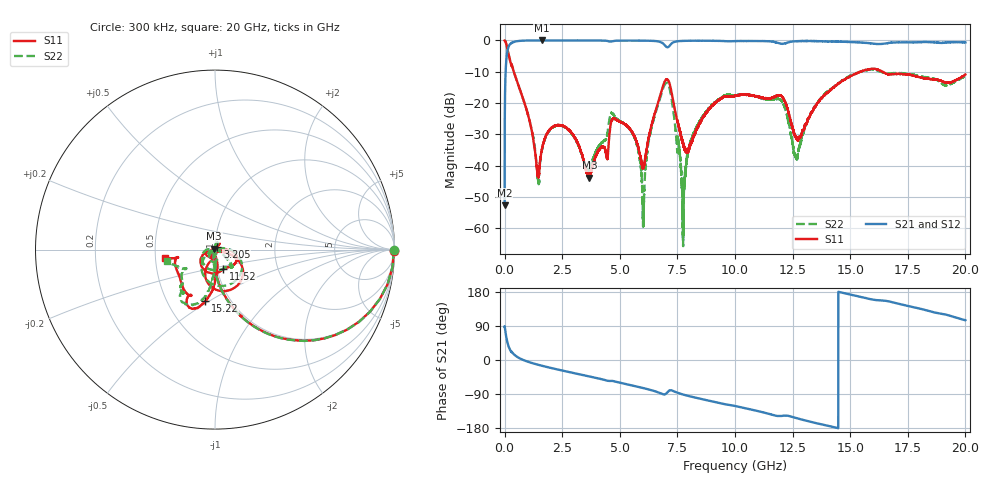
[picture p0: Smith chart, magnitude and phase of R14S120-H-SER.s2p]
!{R14S120}
!Johanson Technology Inc.
!www.johansontechnology.com
!Test Board Conditions:
!Substrate Type  RO4350B
!Substrate Thickness  20 mil
!Substrate Dk  3.66
!TL Type: GCPW
!TL Trace Width  36 mil
!TL Gap  12 mil
!Electrode orientation  Horizontal
!DUT TOPOLOGY	SERIES
!Mounting Pad LxW  26x36 mil
! Created Wed Nov 25 17:33:21 2020
! 2 Port Network Data from SP1.SP block
! freq  magS11  angS11  magS21  angS21  magS12  angS12  magS22  angS22
# khz S ma R 50
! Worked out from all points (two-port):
!   20001 points, 300 kHz to 20 GHz, reference 50 ohm
!   highest |S21| = 0.00 dB at 1.611 GHz (marker M1); lowest = -52.6 dB at 300 kHz (marker M2)
!   |S21| within 3 dB of the highest: 133.4 MHz to end of sweep
!   lowest |S11| = -43.9 dB at 3.683 GHz (marker M3), VSWR 1.01, Z = 49.6 + j0.485 ohm
!   |S11| at or under -10 dB: 400.2 MHz to 15.45 GHz (15.05 GHz wide, 190 % of centre); 15.45674 GHz to 15.4599 GHz (3.157 MHz wide, 0.0204 % of centre); 16.4 GHz to end of sweep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
!   |S22| runs from -65.7 to 0.0 dB; largest |S21 - S12| = 0.019
!   S11 on the Smith chart (normalised r, x): 300 kHz: open; 3.205 GHz: 1.03, +0.03; 11.52 GHz: 1.07, -0.24; 15.22 GHz: 0.77, -0.48; 20 GHz: 0.56, -0.06
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300  0.9967 -0.3  0.002344 88.2  0.002157 90.0  0.9959 -0.3
103300  0.7877 -38.8  0.6122 51.1  0.6139 51.1  0.7882 -38.7
193300  0.5593 -57.4  0.8257 32.3  0.8259 32.2  0.5606 -57.4
1429300  0.007568 -42.7  0.9984 -12.1  0.9986 -12.1  0.007105 -141.8
1611300  0.01771 53.8  0.9996 -15.0  0.9982 -15.0  0.01701 92.6
3205300  0.02158 51.9  0.9975 -37.2  0.9984 -37.2  0.02117 49.2
3334300  0.01599 56.6  0.9977 -38.9  0.9981 -38.9  0.01575 38.0
3683300  0.006403 130.2  0.9975 -43.5  0.9973 -43.5  0.009023 -44.4
4686300  0.0551 -140.0  0.9736 -55.3  0.9755 -55.3  0.06774 -111.3
5624300  0.02984 -159.7  0.9943 -68.5  0.9937 -68.5  0.02908 -144.4
6022300  0.009424 -84.8  0.9911 -74.2  0.9926 -74.2  0.001147 -53.0
6667300  0.1033 -19.0  0.9675 -85.5  0.9666 -85.4  0.09593 -2.8
7147300  0.2125 -94.2  0.8094 -80.6  0.8098 -80.6  0.1782 -103.3
7757300  0.02148 -98.9  0.9845 -91.2  0.9843 -91.3  0.001919 -51.9
8399300  0.04272 -3.6  0.9909 -101.0  0.9894 -101.0  0.04564 -29.7
1.00003e7  0.1297 -23.9  0.9763 -121.3  0.976 -121.4  0.132 -46.4
1.15203e7  0.1188 -66.8  0.9671 -143.0  0.965 -142.9  0.1144 -56.1
1.26413e7  0.02963 -137.0  0.9729 -153.0  0.9746 -153.0  0.01413 -145.0
1.33343e7  0.07251 -79.9  0.9803 -163.8  0.9813 -163.8  0.07246 -87.7
1.52193e7  0.2917 -100.6  0.9367 169.6  0.9405 169.4  0.2953 -105.4
1.66673e7  0.2852 -118.3  0.9121 154.8  0.9054 154.5  0.2946 -125.7
2e7  0.2863 -170.6  0.929 104.9  0.9267 105.1  0.2731 -166.3
